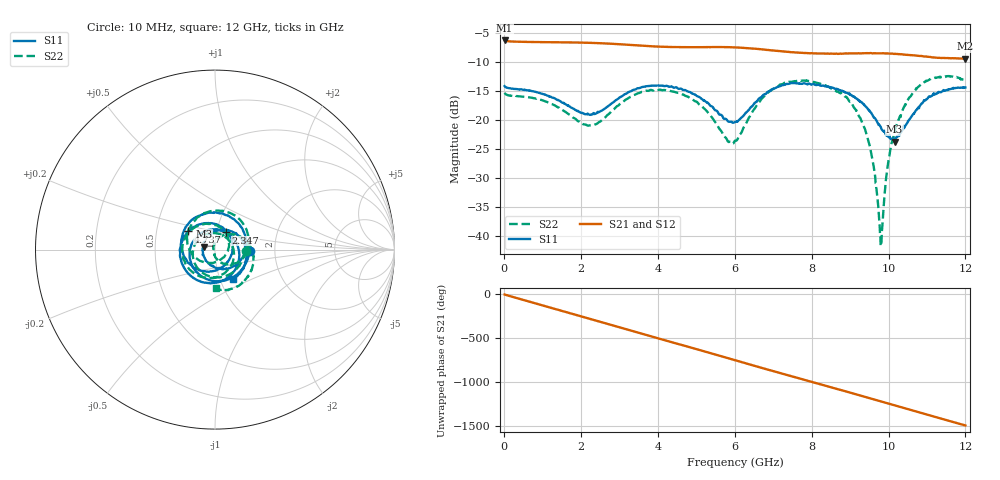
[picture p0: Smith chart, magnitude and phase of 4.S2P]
!Agilent Technologies,E5071C,MY46316741,A.11.02
!Date: Wed Sep 16 11:44:23 2020
!Data & Calibration Information:
!Freq	S11:SOLT2(ON)	S21:SOLT2(ON)	S12:SOLT2(ON)	S22:SOLT2(ON)
!PortZ  Port1:50+j0  Port2:50+j0
!Above PortZ is port z conversion or system Z0 setting when saving the data.
!When reading, reference impedance value at option line is always used.
# Hz S dB R 50
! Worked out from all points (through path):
!   1561 points, 10 MHz to 12 GHz, reference 50 ohm
!   highest |S21| = -6.21 dB at 10 MHz (marker M1); lowest = -9.4 dB at 12 GHz (marker M2)
!   group delay of S21, straight-line fit = 346 ps
!   lowest |S11| = -23.7 dB at 10.16 GHz (marker M3), VSWR 1.14, Z = 44 + j1.52 ohm
!   |S11| at or under -10 dB: start of sweep to end of sweep
!   |S22| runs from -41.7 to -12.4 dB; largest |S21 - S12| = 0.0032
!   S11 on the Smith chart (normalised r, x): 10 MHz: 1.49, -0.02; 2.347 GHz: 1.11, +0.21; 4.737 GHz: 0.73, +0.15; 12 GHz: 1.16, -0.39
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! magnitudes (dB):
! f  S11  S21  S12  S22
! 10 MHz  -14.1  -6.2  -6.2  -15.2
! 1.132 GHz  -15.8  -6.5  -6.5  -16.9
! 2.016 GHz  -18.7  -6.6  -6.6  -20.4
! 2.347 GHz  -18.9  -6.6  -6.6  -20.7
! 3.3 GHz  -15.0  -7.0  -7.0  -15.9
! 4.007 GHz  -14.0  -7.3  -7.3  -14.8
! 4.737 GHz  -14.9  -7.4  -7.4  -15.8
! 6.005 GHz  -20.3  -7.4  -7.4  -23.5
! 6.912 GHz  -14.9  -7.9  -7.9  -14.9
! 8.011 GHz  -13.8  -8.4  -8.4  -13.3
! 8.81 GHz  -15.0  -8.5  -8.5  -15.5
! 9.287 GHz  -16.8  -8.4  -8.4  -20.0
! 9.579 GHz  -19.0  -8.4  -8.4  -26.6
! 9.802 GHz  -21.2  -8.4  -8.5  -41.6
! 9.84 GHz  -21.7  -8.4  -8.4  -38.0
! 9.925 GHz  -22.4  -8.4  -8.4  -30.6
! 10 GHz  -22.8  -8.5  -8.5  -26.8
! 10.16 GHz  -23.7  -8.5  -8.5  -22.0
! 10.48 GHz  -20.5  -8.7  -8.7  -16.7
! 10.87 GHz  -17.0  -8.9  -8.9  -13.6
! 11.54 GHz  -14.7  -9.2  -9.2  -12.4
! 12 GHz  -14.3  -9.4  -9.4  -13.3
